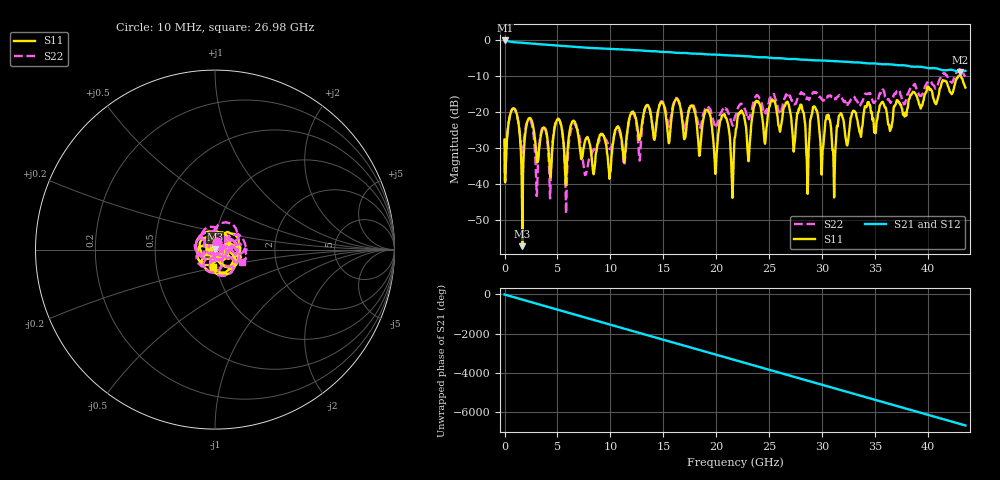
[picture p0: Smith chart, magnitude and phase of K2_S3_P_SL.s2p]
!Keysight Technologies,N5244B,MY57181199,A.13.25.04
!Date: Thursday, May 09, 2019 14:12:10
!Correction: S33(Full 2 Port(3,4))
!S43(Full 2 Port(3,4))
!S34(Full 2 Port(3,4))
!S44(Full 2 Port(3,4))
!S2P File: Measurements: S33, S43, S34, S44:
# Hz S  dB  R 50
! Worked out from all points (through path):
!   4350 points, 10 MHz to 43.5 GHz, reference 50 ohm
!   highest |S21| = -0.05 dB at 20 MHz (marker M1); lowest = -8.8 dB at 42.97 GHz (marker M2)
!   group delay of S21, straight-line fit = 425 ps
!   lowest |S11| = -57.3 dB at 1.68 GHz (marker M3), VSWR 1.00, Z = 50.1 + j0.124 ohm
!   |S11| at or under -10 dB: start of sweep to 42.83 GHz; 43.08 GHz to end of sweep
!   |S22| runs from -48.3 to -8.0 dB; largest |S21 - S12| = 0.00089
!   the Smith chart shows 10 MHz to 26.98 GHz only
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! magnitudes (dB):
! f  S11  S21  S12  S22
! 10 MHz  -27.6  -0.1  -0.1  -27.6
! 20 MHz  -33.3  0.0  0.0  -33.5
! 940 MHz  -19.1  -0.5  -0.5  -19.2
! 1.68 GHz  -57.3  -0.7  -0.7  -31.4
! 2.36 GHz  -21.6  -0.9  -0.9  -22.0
! 3.04 GHz  -32.7  -1.0  -1.0  -43.4
! 5.01 GHz  -22.1  -1.5  -1.5  -21.9
! 5.8 GHz  -40.2  -1.6  -1.6  -47.2
! 6.46 GHz  -22.4  -1.8  -1.8  -23.5
! 7.26 GHz  -33.1  -2.0  -2.0  -30.6
! 14.51 GHz  -19.5  -3.1  -3.1  -19.4
! 21.76 GHz  -26.9  -4.3  -4.3  -21.4
! 25.33 GHz  -17.0  -5.0  -5.0  -15.4
! 27.31 GHz  -30.7  -5.2  -5.2  -17.8
! 28.06 GHz  -18.5  -5.4  -5.4  -14.8
! 28.61 GHz  -42.7  -5.4  -5.4  -16.1
! 29.01 GHz  -20.6  -5.5  -5.5  -15.2
! 31.09 GHz  -41.5  -5.8  -5.8  -16.4
! 31.71 GHz  -20.4  -5.9  -5.9  -15.7
! 36.26 GHz  -23.4  -6.7  -6.7  -16.4
! 42.97 GHz  -9.8  -8.8  -8.8  -8.0
! 43.5 GHz  -13.1  -8.5  -8.5  -10.1
